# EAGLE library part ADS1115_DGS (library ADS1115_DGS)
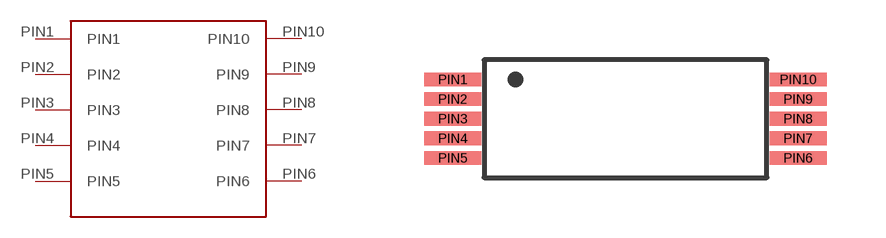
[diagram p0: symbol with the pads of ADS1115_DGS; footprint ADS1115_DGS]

Designator prefix -

## ADS1115_DGS  [ADS1115_DGS]
PIN1  PIN1
PIN2  PIN2
PIN3  PIN3
PIN4  PIN4
PIN5  PIN5
PIN6  PIN6
PIN7  PIN7
PIN8  PIN8
PIN9  PIN9
PIN10  PIN10

## Footprint ADS1115_DGS (pad centres in mm)
smd 1.45 x 0.35: PIN1 -4.4,1; PIN2 -4.4,0.5; PIN3 -4.4,0; PIN4 -4.4,-0.5; PIN5 -4.4,-1; PIN6 4.4,-1; PIN7 4.4,-0.5; PIN8 4.4,0; PIN9 4.4,0.5; PIN10 4.4,1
